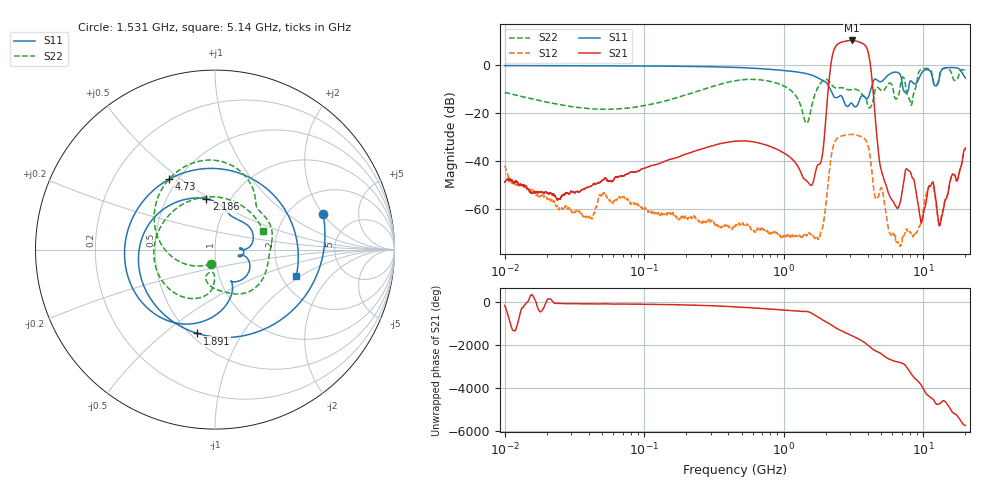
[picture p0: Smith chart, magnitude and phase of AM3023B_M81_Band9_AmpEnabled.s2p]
!Agilent Technologies,E8364B,MY43040894,A.07.50.67
!Agilent E8364B: A.07.50.67
!Date: Tuesday, October 27, 2020 10:45:01
!Correction: S11(Full 2 Port(1,2))
!S21(Full 2 Port(1,2))
!S12(Full 2 Port(1,2))
!S22(Full 2 Port(1,2))
!S2P File: Measurements: S11, S21, S12, S22:Log Frequency Sweep
# Hz S  dB  R 50
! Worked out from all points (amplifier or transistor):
!   3201 points, 10 MHz to 20 GHz, reference 50 ohm
!   highest |S21| = 10.2 dB at 3.077 GHz (marker M1)
!   |S21| within 3 dB of that: 2.326 GHz to 3.924 GHz (1.598 GHz wide, 51.2 % of centre)
!   unconditionally stable (mu >= 1): start of sweep to end of sweep
!   at 35.47 MHz: K = 19938.32, MAG = -41.1 dB, |S12| = -61.9 dB
!   at 447.2 MHz: K = 7328.85, MAG = -23.9 dB, |S12| = -67.4 dB
!   at 20 GHz: K = 449.67, MAG = -29.3 dB, |S12| = -35.1 dB
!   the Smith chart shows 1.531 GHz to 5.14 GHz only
!   S11 on the Smith chart (normalised r, x): 1.531 GHz: 3.02, +2.01; 1.891 GHz: 0.54, -0.66; 2.186 GHz: 0.78, +0.48; 4.73 GHz: 0.45, +0.45; 5.14 GHz: 2.42, -0.91
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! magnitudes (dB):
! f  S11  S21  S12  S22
! 10 MHz  -0.3  -48.7  -42.0  -11.6
! 35.55 MHz  -0.4  -52.0  -61.9  -17.9
! 51.38 MHz  -0.4  -47.8  -53.3  -18.5
! 126.1 MHz  -0.5  -41.2  -61.7  -15.7
! 447.2 MHz  -1.0  -31.8  -67.4  -6.6
! 988.7 MHz  -2.3  -36.5  -71.5  -8.6
! 1.531 GHz  -4.0  -49.8  -70.4  -21.4
! 1.59 GHz  -4.3  -50.1  -70.8  -16.8
! 1.891 GHz  -6.4  -37.4  -67.8  -6.8
! 2.186 GHz  -10.9  1.0  -38.1  -8.0
! 3.077 GHz  -16.0  10.2  -29.0  -10.3
! 4.015 GHz  -13.6  5.5  -33.7  -17.3
! 4.73 GHz  -6.6  -34.5  -55.2  -9.4
! 5.14 GHz  -6.4  -46.4  -53.6  -10.8
! 5.639 GHz  -4.1  -53.7  -68.8  -7.7
! 6.612 GHz  -3.2  -59.5  -74.4  -13.0
! 7.679 GHz  -11.3  -43.5  -69.0  -12.5
! 8.709 GHz  -7.9  -50.2  -70.8  -10.3
! 9.692 GHz  -3.5  -65.8  -65.0  -1.8
! 11.26 GHz  -2.8  -50.4  -50.8  -2.2
! 13.17 GHz  -3.8  -66.8  -65.5  -3.2
! 20 GHz  -5.4  -34.6  -35.1  -2.3
